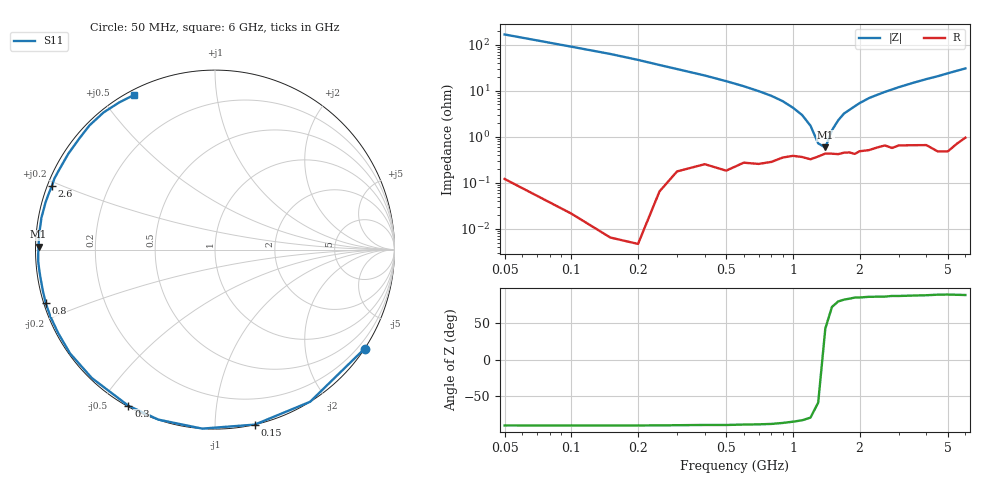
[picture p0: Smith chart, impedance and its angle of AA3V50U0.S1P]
! Infineon Technologies  Discrete & RF Semiconductors
! BBY66-02W
! Si Tuning Diode in SCD-80
! VR = 3.5 V
! S-Parameters:  June  2000
# GHz  S  MA  R  50
!  f  S11
! GHz  MAG  ANG
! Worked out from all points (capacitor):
!   34 points, 50 MHz to 6 GHz, reference 50 ohm
!   read as one part to ground: C = 17.5 pF near 50 MHz
!   lowest |Z| = 581 mohm at 1.4 GHz (marker M1)
!   series resonance near 1.361 GHz, so ESL is about 780 pH
!   S11 on the Smith chart (normalised r, x): 50 MHz: 0.00, -3.32; 150 MHz: 0.00, -1.25; 300 MHz: 0.00, -0.59; 800 MHz: 0.01, -0.15; 2.6 GHz: 0.01, +0.19; 6 GHz: 0.02, +0.61
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0.05  0.9996 -33.5
0.1  0.9998 -58.0
0.15  0.9999 -77.2
0.2  0.9999 -94.1
0.25  0.9983 -108.4
0.3  0.9948 -119.0
0.4  0.9915 -133.8
0.5  0.9934 -144.4
0.6  0.9898 -152.0
0.7  0.9902 -157.9
0.8  0.989 -162.5
1  0.9849 -170.3
1.2  0.9872 -176.1
1.4  0.983 179.1
1.6  0.9835 174.9
1.7  0.9823 172.8
1.9  0.9834 169.6
2.2  0.9802 164.4
2.4  0.9776 161.6
2.6  0.9754 158.8
2.8  0.9785 156.1
3  0.9759 153.3
3.5  0.9763 146.9
4  0.977 140.8
4.5  0.9838 135.3
5  0.9845 129.1
5.5  0.9784 123.1
6  0.9726 117.5
